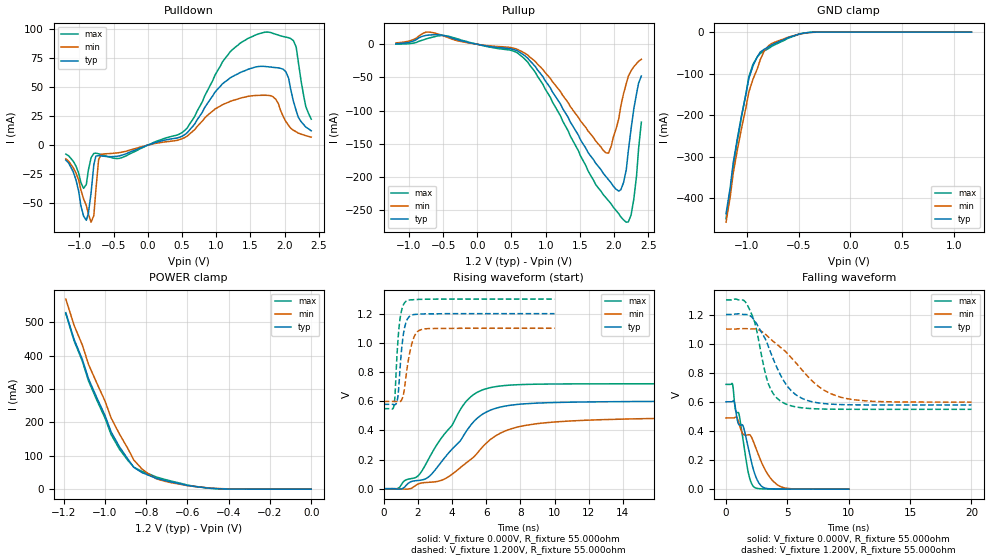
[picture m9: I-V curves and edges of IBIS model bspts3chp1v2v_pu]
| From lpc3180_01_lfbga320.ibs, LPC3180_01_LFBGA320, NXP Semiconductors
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| |   Rev 0.20 IBIS Model Design Automation Generation   |
| |   N O N - S I L I C O N   C O R R E L A T E D   |
| |   This IBIS [Model] is pre-Beta tactical support   |
| |  Note: this IBIS [Model] contains clamp curves generated   |
| |   through simulation which should not be relied upon   |
| bspts3chp1v2v
|   Bidirectional Pad 1v2
|   3state Output
|   Plain Input
|   3ns Slew Rate control
|   CMOS
|   Programmable between
|   - (p1=0, p2=1) plain input
|   - (p1=0, p2=0) with Pull Up
|   - (p1=1, p2=1) with Pull Down
|   - (p1=1, p2=0) with Repeater
|   Characterized at Core 1.2V and I/O 1.2V
| Pull Up Mode (p1=0, p2=0)
[Model]   bspts3chp1v2v_pu | of bspts3chp1v2v
Model_type   I/O
Polarity   Non-Inverting
Enable   Active-Low
|  Reciever Thresholds
Vinl   = 0.36V
Vinh   = 0.84V
| AC Test Load Conditions
Vref   = 0
Cref   = 1.2e-11
Rref   = 1000000000
Vmeas   = 0.6
| [Process Range]   typical   min   max
| C_comp edge width   400.000ps   400.000ps   400.000ps
| C_comp Tstrobe   40.000fs   40.000fs   40.000fs
C_comp   2.975pF   2.770pF   3.253pF
[Temperature Range]   25   105   -20
[Voltage Range]   1.20V   1.10V   1.30V
[GND Clamp Reference]   0.00V   0.00V   0.00V
[Pulldown Reference]   0.00V   0.00V   0.00V
[POWER Clamp Reference]   1.20V   1.10V   1.30V
[Pullup Reference]   1.20V   1.10V   1.30V
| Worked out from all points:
|   slope of the pulldown table from 0 to 0.18 V, typ, clamps not added: 55.1 ohm
|   slope of the pullup table from 0 to 0.18 V, typ, clamps not added: 53.4 ohm
|   GND clamp passes 1 mA (typ) near -0.40 V on its own axis
|   POWER clamp passes 1 mA (typ) near -0.43 V on its own axis
|   rising waveform, V_fixture 0.000V, R_fixture 55.000ohm: 20-80 % time 2.49ns typ, 3ns min, 2.33ns max; typ from 0.001 V to 0.6 V
|   falling waveform, V_fixture 0.000V, R_fixture 55.000ohm: 20-80 % time 1.38ns typ, 2.14ns min, 1.03ns max; typ from 0.601 V to 0.001 V
|   rising waveform, V_fixture 1.200V, R_fixture 55.000ohm: 20-80 % time 290ps typ, 433ps min, 251ps max; typ from 0.579 V to 1.2 V
|   falling waveform, V_fixture 1.200V, R_fixture 55.000ohm: 20-80 % time 2.13ns typ, 3.58ns min, 1.25ns max; typ from 1.2 V to 0.579 V
[GND Clamp]
| ref voltage   0.00V   0.00V   0.00V
|   Voltage   I(typ)   I(min)   I(max)
-1.2V     -437mA     -457.3mA   -448.8mA
-1.16V    -374mA     -396.6mA   -383.9mA
-1.13V    -313.1mA   -338.2mA   -320.9mA
-1.05V    -200.5mA   -230.7mA   -202.9mA
-980mV    -111.6mA   -144.4mA   -108mA
-940mV    -81.37mA   -113.4mA   -77.55mA
-870mV    -48.12mA   -66.68mA   -51.41mA
-830mV    -41.11mA   -44.63mA   -45.12mA
-790mV    -35.73mA   -33.03mA   -39.62mA
-570mV    -10.71mA   -10.12mA   -11.96mA
-390mV    -633uA     -1.091mA   -535.9uA
1.17V     -2.05uA    3.702uA    -9.85uA
[Power Clamp]   | Vtable = Vcc - Vpad
| ref voltage   1.20V   1.10V   1.30V
|   Voltage   I(typ)   I(min)   I(max)
-1.19V    529.3mA    570.1mA    526.5mA
-1.15V    449.5mA    491.7mA    445.3mA
-1.11V    389.5mA    432.5mA    384.2mA
-1.08V    331.1mA    374.7mA    324.8mA
-1V       221.2mA    264.5mA    213.3mA
-970mV    171.4mA    213.2mA    163.4mA
-890mV    91.03mA    122.9mA    86.98mA
-860mV    65.38mA    87.23mA    65.77mA
-820mV    49.53mA    60.17mA    53.08mA
-750mV    32.1mA     30.88mA    36.28mA
-560mV    7.554mA    7.588mA    8.109mA
0V        329.3nA    291.4nA    400.7nA
[Pulldown]
| ref voltage   0.00V   0.00V   0.00V
|   Voltage   I(typ)   I(min)   I(max)
-1.2V     -12.9mA    -11.81mA   -7.732mA
-900mV    -64.77mA   -51.94mA   -33.88mA
-830mV    -40.99mA   -66.41mA   -10.77mA
-760mV    -9.399mA   -38.71mA   -6.922mA
-720mV    -9.108mA   -12.33mA   -7.471mA
-680mV    -9.342mA   -7.831mA   -8.122mA
500mV     7.668mA    5.475mA    10.77mA
1.2V      57.8mA     37.61mA    80.16mA
1.72V     67.75mA    42.97mA    97.43mA
2.02V     63.13mA    20.22mA    93.1mA
2.13V     37.64mA    12.84mA    90mA
2.39V     12.34mA    6.89mA     22.38mA
[Pullup]   | Vtable = Vcc - Vpad
| ref voltage   1.20V   1.10V   1.30V
|   Voltage   I(typ)   I(min)   I(max)
-1.19V    982.9uA    2.112mA    262.9uA
-710mV    13.91mA    18.44mA    9.272mA
-450mV    12.25mA    11.02mA    12.78mA
590mV     -9.984mA   -7.698mA   -13.1mA
960mV     -48.83mA   -37.98mA   -60.41mA
1.88V     -199.3mA   -163.7mA   -231.3mA
1.96V     -209.3mA   -153.4mA   -241mA
2.07V     -221.5mA   -112.2mA   -255.7mA
2.18V     -188.7mA   -59.17mA   -268.4mA
2.25V     -127.4mA   -39.92mA   -257.5mA
2.33V     -74.26mA   -29.16mA   -198.1mA
2.4V      -47.76mA   -22.65mA   -117.4mA
[Ramp]
R_load   = 55.000ohm
|   dV/dt(typ)   dV/dt(min)   dV/dt(max)
dV/dt_r   337.907mV/2.450ns   259.224mV/2.715ns   412.702mV/2.315ns
dV/dt_f   356.319mV/2.195ns   272.300mV/3.335ns   433.855mV/1.325ns
[Rising Waveform]  | cubic spline decimation from 4001 points
V_fixture   = 0.000V
R_fixture   = 55.000ohm
|   Time   V(typ)   V(min)   V(max)
0s        608.3uV    506.1uV    731.7uV
755ps     -598.5uV   817.1uV    -1.561mV
1.915ns   56.03mV    26.23mV    80.21mV
2.6ns     78.7mV     44.2mV     197.5mV
3.555ns   210.7mV    66.41mV    374.9mV
4.795ns   386.5mV    173.9mV    594.1mV
5.95ns    522.4mV    306.6mV    684.1mV
7.09ns    566.4mV    395.4mV    707.6mV
9.25ns    588.4mV    449.9mV    717.2mV
20ns      600mV      486.6mV    720mV
[Falling Waveform]  | cubic spline decimation from 2001 points
V_fixture   = 0.000V
R_fixture   = 55.000ohm
|   Time   V(typ)   V(min)   V(max)
0s        600.9mV    489.9mV    720.1mV
525ps     602.4mV    490mV      722.6mV
755ps     563.3mV    494.8mV    549.7mV
1.055ns   443.2mV    452.3mV    516.7mV
1.4ns     432.6mV    377.9mV    332.3mV
1.815ns   283.4mV    374.3mV    113.7mV
2.29ns    118.1mV    313.8mV    14.73mV
3.02ns    13.3mV     160.4mV    2.551mV
4.305ns   1.583mV    23.82mV    1.086mV
10ns      616.2uV    598uV      733.2uV
[Rising Waveform]  | cubic spline decimation from 2001 points
V_fixture   = 1.200V
V_fixture_min = 1.100V
V_fixture_max = 1.300V
R_fixture   = 55.000ohm
|   Time   V(typ)   V(min)   V(max)
0s        578.8mV    598.5mV    549mV
600ps     577.2mV    598.5mV    567.7mV
670ps     576.5mV    598.5mV    651.5mV
800ps     607.5mV    597mV      950.3mV
925ps     765.2mV    596.4mV    1.134V
1.12ns    1.029V     628.5mV    1.251V
1.315ns   1.142V     775.9mV    1.285V
1.7ns     1.192V     1.014V     1.295V
2.16ns    1.198V     1.089V     1.298V
10ns      1.2V       1.1V       1.3V
[Falling Waveform]  | cubic spline decimation from 4001 points
V_fixture   = 1.200V
V_fixture_min = 1.100V
V_fixture_max = 1.300V
R_fixture   = 55.000ohm
|   Time   V(typ)   V(min)   V(max)
0s        1.2V       1.1V       1.3V
1.4ns     1.2V       1.103V     1.299V
1.77ns    1.199V     1.102V     1.26V
2.335ns   1.157V     1.101V     1.147V
3.47ns    975.6mV    1.044V     719.6mV
3.995ns   864.3mV    1.005V     639.7mV
4.84ns    726.2mV    946.4mV    586.6mV
6.435ns   615.3mV    795.8mV    557.1mV
9.275ns   581.7mV    633.3mV    549.3mV
20ns      578.8mV    598.5mV    549mV
